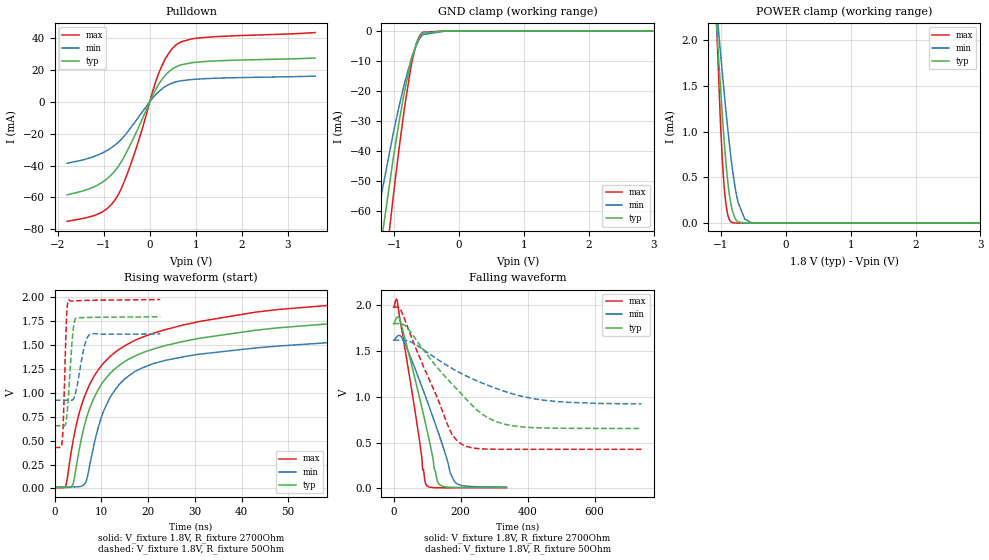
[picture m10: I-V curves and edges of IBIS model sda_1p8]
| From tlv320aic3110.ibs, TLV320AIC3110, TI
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|   sda_1p8 Model
[Model]   sda_1p8
Model_type   I/O_open_drain
Polarity   Inverting
Vinl = 0.54
Vinh = 1.26
Vmeas = 0.9
Vref = 1.8
Cref = 110pF
Rref = 2700
|   typ   min   max
|   (nom PVT)   (fast PVT)   (slow PVT)
C_comp   1.252e-12   1.236e-12   1.258e-12
[Model spec]
Vinl   0.54   0.486   0.594
Vinh   1.26   1.134   1.386
| Where nom  PVT is Nominal Process, 1.8V, 27C
|   Fast PVT is Strong Process,  1.98V, -40C
|   Slow PVT is Weak Process,   1.62V, 125C
[Voltage Range]   1.8   1.62   1.98
|Junction Temperature
[Temperature Range]   27   125   -40
[Pullup Reference]   1.8   1.62   1.98
[Pulldown Reference]   0   0   0
[Power Clamp Reference]   1.8   1.62   1.98
[GND Clamp Reference]   0   0   0
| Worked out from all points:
|   slope of the pulldown table from 0 to 0.27 V, typ, clamps not added: 19 ohm
|   GND clamp passes 1 mA (typ) near -0.57 V on its own axis
|   POWER clamp passes 1 mA (typ) near -0.96 V on its own axis
|   falling waveform, V_fixture 1.8V, R_fixture 2700Ohm: 20-80 % time 67.8ns typ, 92.9ns min, 50.6ns max; typ from 1.8 V to 0.01 V
|   rising waveform, V_fixture 1.8V, R_fixture 2700Ohm: 20-80 % time 15ns typ, 12.8ns min, 15.4ns max; typ from 0.01 V to 1.8 V
|   falling waveform, V_fixture 1.8V, R_fixture 50Ohm: 20-80 % time 163ns typ, 227ns min, 105ns max; typ from 1.8 V to 0.656 V
|   rising waveform, V_fixture 1.8V, R_fixture 50Ohm: 20-80 % time 952ps typ, 1.57ns min, 575ps max; typ from 0.656 V to 1.8 V
[Pulldown]
|   Voltage   I(typ)   I(min)   I(max)
-1.8V     -58.41mA   -38.57mA   -74.97mA
-1.054V   -50.86mA   -32.42mA   -69.37mA
-847.8mV  -46.1mA    -29.07mA   -64.78mA
-707.4mV  -41.4mA    -25.97mA   -59.29mA
-574.4mV  -35.36mA   -22.11mA   -51.37mA
-366.3mV  -23.53mA   -14.43mA   -35.19mA
66.24mV   4.23mA     2.417mA    6.876mA
193.9mV   10.97mA    6.294mA    17.77mA
358.2mV   17.22mA    9.881mA    27.9mA
570.6mV   21.88mA    12.46mA    35.58mA
1.115V    25.03mA    14.32mA    40.1mA
3.6V      27.37mA    16.02mA    43.36mA
[GND Clamp]
|   Voltage   I(typ)   I(min)   I(max)
-1.8V     -265.1mA   -154.4mA   -381.7mA
-1.349V   -93.56mA   -71.94mA   -120mA
-1.252V   -78.05mA   -60.45mA   -100.7mA
-1.016V   -42.44mA   -34.1mA    -55.13mA
-920.3mV  -29.65mA   -24.57mA   -38.23mA
-859.5mV  -22.23mA   -18.98mA   -28.29mA
-747mV    -10.58mA   -9.981mA   -12.55mA
-657.5mV  -4.082mA   -4.619mA   -4.078mA
-606.1mV  -1.843mA   -2.515mA   -1.515mA
-558mV    -715.8uA   -1.245mA   -464.5uA
-180mV    0A         -211.6nA   0A
3.6V      0A         0A         0A
[POWER Clamp]
|   Voltage   I(typ)   I(min)   I(max)
-1.8V     11.74mA    8.748mA    19.35mA
-1.075V   2.291mA    2.431mA    2.403mA
-1.058V   2.089mA    2.292mA    2.061mA
-1.004V   1.481mA    1.865mA    1.095mA
-972.4mV  1.145mA    1.619mA    648.1uA
-948.6mV  911.8uA    1.439mA    403.5uA
-901.8mV  521.3uA    1.1mA      123.2uA
-835.2mV  180.5uA    670.8uA    9.313uA
-732.4mV  12.01uA    226.7uA    83.67nA
-630.4mV  330.9nA    44.02uA    0A
-528.3mV  0A         3.711uA    0A
3.6V      0A         0A         0A
[Ramp]
R_load = 2700
|   typ   min   max
dV/dt_r   1.07409/1.49537e-08   0.962648/1.28059e-08   1.18401/1.53565e-08
dV/dt_f   1.07409/6.79996e-08   0.962648/9.29657e-08   1.18401/5.06373e-08
[Falling Waveform]
V_fixture = 1.8V
V_fixture_min = 1.62V
V_fixture_max = 1.98V
R_fixture = 2700Ohm
|   Time   V(typ)   V(min)   V(max)
0s        1.8V       1.62V      1.98V
11.08ns   1.873V     1.665V     2.04V
30.58ns   1.679V     1.608V     1.597V
74.14ns   1.039V     1.21V      596.4mV
86.62ns   844.2mV    1.088V     203.9mV
95.68ns   699.7mV    998.1mV    48.02mV
132ns     66.91mV    623.3mV    7.698mV
168.5ns   13.44mV    173.3mV    6.699mV
183.2ns   11.82mV    69.73mV    6.582mV
336.5ns   9.783mV    15.6mV     6.644mV
[Rising Waveform]
V_fixture = 1.8V
V_fixture_min = 1.62V
V_fixture_max = 1.98V
R_fixture = 2700Ohm
|   Time   V(typ)   V(min)   V(max)
0s        9.857mV    15.58mV    6.645mV
2.32ns    9.467mV    15.58mV    19.96mV
3.94ns    47.85mV    15.45mV    502mV
6.66ns    714.1mV    65.18mV    996.9mV
9.3ns     1.033V     636.9mV    1.239V
12.02ns   1.212V     967.7mV    1.387V
21.02ns   1.456V     1.305V     1.622V
42.86ns   1.654V     1.469V     1.843V
91.92ns   1.781V     1.587V     1.967V
243.6ns   1.8V       1.62V      1.98V
[Falling Waveform]
V_fixture = 1.8V
V_fixture_min = 1.62V
V_fixture_max = 1.98V
R_fixture = 50Ohm
|   Time   V(typ)   V(min)   V(max)
0s        1.8V       1.62V      1.98V
22.26ns   1.8V       1.621V     1.941V
36.38ns   1.771V     1.617V     1.814V
61.2ns    1.655V     1.582V     1.578V
174.1ns   1.142V     1.312V     582mV
203.6ns   1.027V     1.253V     481.5mV
263.1ns   815.3mV    1.153V     432.7mV
345ns     690.9mV    1.044V     427.9mV
482.6ns   658mV      950.8mV    427.7mV
739.9ns   655.6mV    923.6mV    427.7mV
[Rising Waveform]
V_fixture = 1.8V
V_fixture_min = 1.62V
V_fixture_max = 1.98V
R_fixture = 50Ohm
|   Time   V(typ)   V(min)   V(max)
0s        655.6mV    922.9mV    427.7mV
1.6ns     655.5mV    922.9mV    499.4mV
1.86ns    655mV      922.9mV    742.2mV
2.54ns    740.6mV    923mV      1.806V
3ns       1.017V     922.6mV    1.972V
3.8ns     1.589V     925.7mV    1.96V
4.52ns    1.781V     1.013V     1.963V
6.12ns    1.788V     1.441V     1.966V
7.32ns    1.789V     1.605V     1.967V
22.6ns    1.797V     1.617V     1.977V
